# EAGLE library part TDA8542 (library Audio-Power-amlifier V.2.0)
2 ´ 1 W BTL audio amplifier
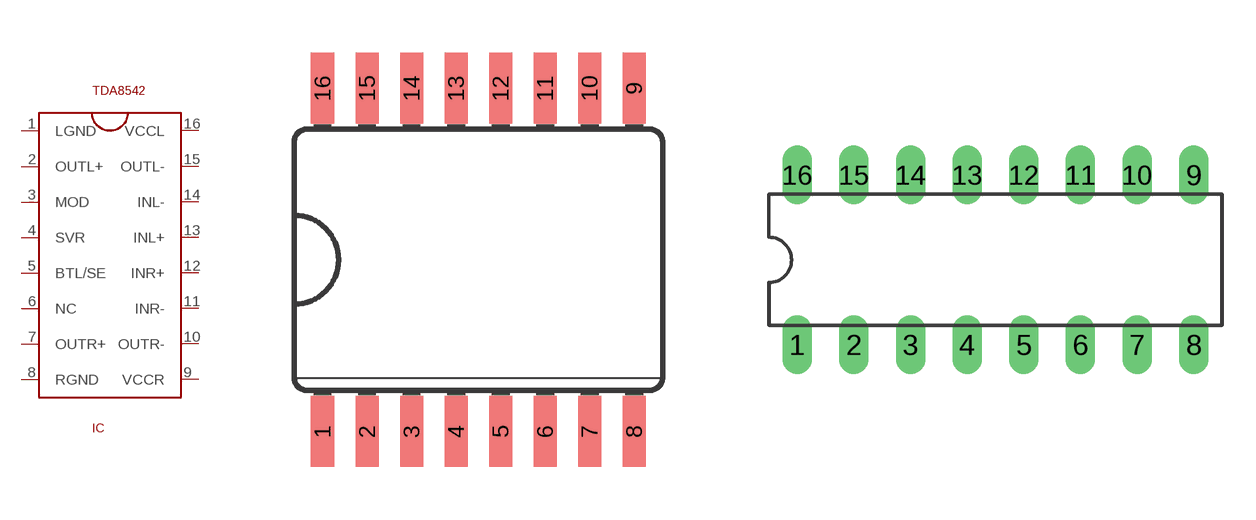
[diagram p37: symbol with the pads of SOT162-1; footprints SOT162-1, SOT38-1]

Designator prefix IC

## TDA8542  [SOT162-1]
1  LGND  pwr
2  OUTL+  out
3  MOD
4  SVR
5  BTL/SE
6  NC  nc
7  OUTR+  out
8  RGND  pwr
9  VCCR  pwr
10  OUTR-  out
11  INR-  in
12  INR+  in
13  INL+  in
14  INL-  in
15  OUTL-  out
16  VCCL  pwr

## TDA8542SOT38-1  [SOT38-1]
Pads as for SOT162-1

## Footprint SOT162-1 (pad centres in mm)
Small Outline Package
smd 0.66 x 2.032: 1 -4.445,-4.902; 2 -3.175,-4.902; 3 -1.905,-4.902; 4 -0.635,-4.902; 5 0.635,-4.902; 6 1.905,-4.902; 7 3.175,-4.902; 8 4.445,-4.902; 9 4.445,4.902; 10 3.175,4.902; 11 1.905,4.902; 12 0.635,4.902; 13 -0.635,4.902; 14 -1.905,4.902; 15 -3.175,4.902; 16 -4.445,4.902

## Footprint SOT38-1 (pad centres in mm)
Dual In Line Package
drill 0.813 long: 1 -8.89,-3.81; 2 -6.35,-3.81; 3 -3.81,-3.81; 4 -1.27,-3.81; 5 1.27,-3.81; 6 3.81,-3.81; 7 6.35,-3.81; 8 8.89,-3.81; 9 8.89,3.81; 10 6.35,3.81; 11 3.81,3.81; 12 1.27,3.81; 13 -1.27,3.81; 14 -3.81,3.81; 15 -6.35,3.81; 16 -8.89,3.81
